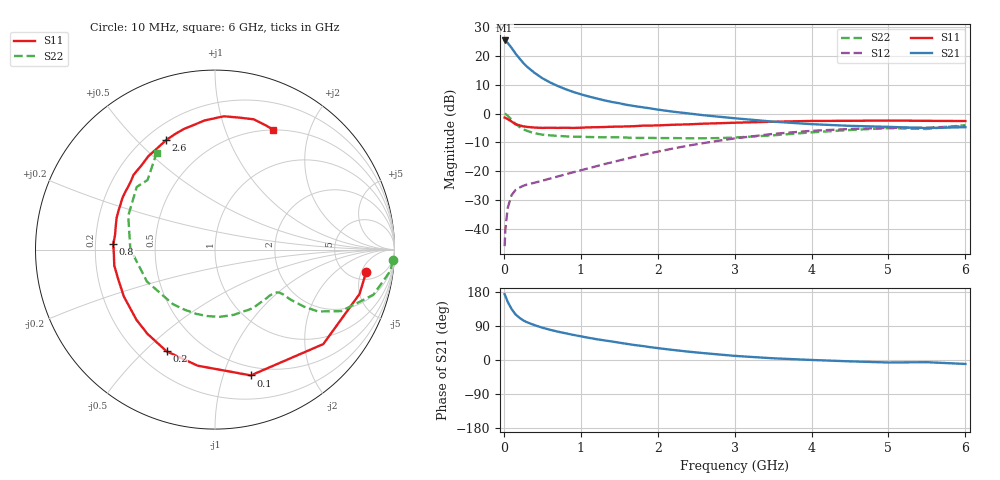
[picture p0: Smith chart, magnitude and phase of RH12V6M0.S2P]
! SIEMENS Small Signal Semiconductors
! BFR106
! Si NPN RF Bipolar Junction Transistor in SOT23
! VCE = 12 V  IC = 6 mA
! Common Emitter S-Parameters:  August  1996
# GHz  S  MA  R  50
!  f  S11  S21  S12  S22
! GHz  MAG  ANG  MAG  ANG  MAG  ANG  MAG  ANG
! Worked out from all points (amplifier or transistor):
!   36 points, 10 MHz to 6 GHz, reference 50 ohm
!   highest |S21| = 25.4 dB at 10 MHz (marker M1)
!   |S21| within 3 dB of that: start of sweep to 111.7 MHz
!   unconditionally stable (mu >= 1): 607.6 MHz to 1.858 GHz; 5.139 GHz to end of sweep
!   at 250 MHz: K = 0.55, MSG = 21.4 dB, |S12| = -25.1 dB
!   at 1.4 GHz: K = 1.12, MAG = 8.4 dB, |S12| = -16.9 dB
!   at 6 GHz: K = 1.01, MAG = -0.9 dB, |S12| = -4.3 dB
!   S11 on the Smith chart (normalised r, x): 10 MHz: 6.67, -6.17; 100 MHz: 0.41, -1.24; 200 MHz: 0.31, -0.59; 800 MHz: 0.28, +0.03; 2.6 GHz: 0.28, +0.61; 6 GHz: 0.50, +1.48
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0.01  0.8513 -8.6  18.55 173.7  0.005 88.2  0.9923 -3.5
0.02  0.8423 -17.1  18.23 169.1  0.0098 77.8  0.9846 -6.9
0.05  0.8007 -41.1  16.81 153.5  0.023 69.3  0.9178 -15.9
0.1  0.7288 -74.1  13.84 134.8  0.0383 55.9  0.7823 -26.0
0.15  0.654 -98.5  11.08 120.7  0.0469 47.9  0.6689 -31.0
0.2  0.6275 -115.5  9.151 112.0  0.0516 44.7  0.5916 -32.6
0.25  0.6015 -128.8  7.622 104.8  0.0556 42.5  0.5347 -33.2
0.3  0.587 -138.2  6.525 99.7  0.0587 42.7  0.5014 -33.5
0.4  0.5711 -152.7  5.074 91.9  0.0631 43.9  0.4548 -33.3
0.5  0.564 -162.7  4.11 85.3  0.0684 46.5  0.4307 -33.7
0.6  0.5683 -171.0  3.47 79.8  0.0744 49.3  0.4189 -34.8
0.8  0.5677 176.9  2.656 70.6  0.088 54.6  0.4027 -38.4
1.1  0.5761 162.1  1.985 58.7  0.1123 60.8  0.3919 -46.0
1.3  0.5838 154.3  1.704 51.9  0.1321 63.3  0.3877 -51.8
1.6  0.598 143.7  1.414 42.5  0.1653 64.9  0.3828 -62.0
2.2  0.6393 125.5  1.078 26.5  0.2475 62.4  0.3755 -86.4
2.6  0.6679 114.1  0.934 18.1  0.3078 57.6  0.373 -106.0
3.5  0.7217 94.6  0.724 4.5  0.444 42.4  0.4191 -155.0
4.5  0.7484 78.9  0.612 -3.6  0.5396 22.6  0.5189 158.7
5  0.7574 73.4  0.588 -6.6  0.5639 14.0  0.5586 141.3
5.5  0.7475 67.5  0.559 -5.8  0.5696 9.5  0.5399 134.1
6  0.7422 64.1  0.58 -10.4  0.6069 1.2  0.6305 121.0
